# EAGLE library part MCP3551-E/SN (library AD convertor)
MCP3551-E/SN AD converter (22bit , SPI interface) 2.7V , ?-? type ADC Producted by Microchip.Co
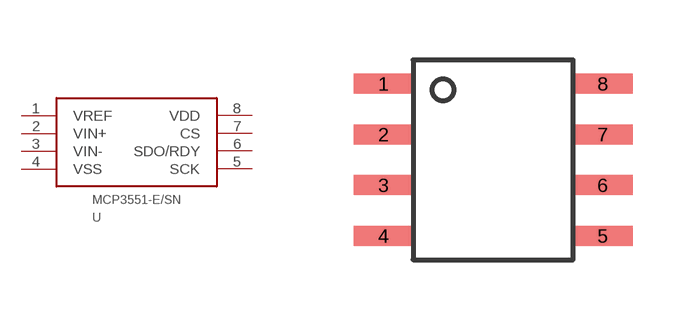
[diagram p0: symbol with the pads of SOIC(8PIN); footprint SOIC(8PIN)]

Designator prefix U

## MCP3551-E/SN  [SOIC(8PIN)]
1  VREF
2  VIN+
3  VIN-
4  VSS
5  SCK
6  SDO/RDY
7  CS
8  VDD

## Footprint SOIC(8PIN) (pad centres in mm)
4*5mm size , 0.05inch pitch , 8pin pacage
smd 1.5 x 0.5: 1 -2.73,1.905; 2 -2.73,0.635; 3 -2.73,-0.635; 4 -2.73,-1.905; 5 2.75,-1.905; 6 2.75,-0.635; 7 2.75,0.635; 8 2.75,1.905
